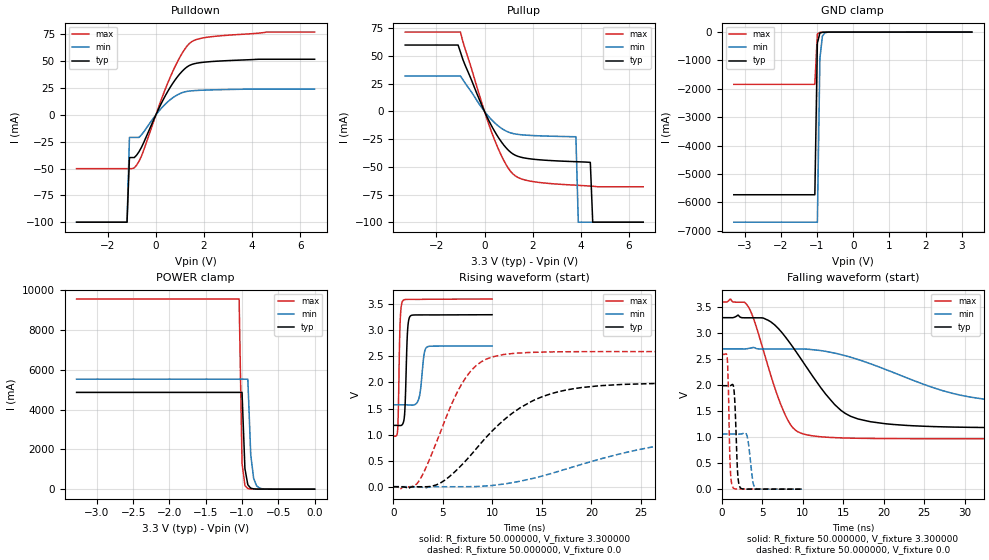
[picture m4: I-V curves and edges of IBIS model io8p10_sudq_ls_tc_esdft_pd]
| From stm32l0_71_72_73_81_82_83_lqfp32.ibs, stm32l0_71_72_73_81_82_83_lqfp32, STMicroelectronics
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|   Model io8p10_sudq_ls_tc_esdft_pd
[Model]  io8p10_sudq_ls_tc_esdft_pd
Model_type I/O
Polarity   Non-Inverting
Enable   Active-Low
Vinl =   0.990000V
Vinh =   2.310000V
Vmeas =  1.650000V
Cref =   50.000000pF
Rref =   100.000000M
Vref =   0.0V
C_comp   2.248300pF   2.207300pF   2.311900pF
[Temperature Range]   25.000000   0.125000k   -40.000000
[Pullup Reference]   3.300000V   2.700000V   3.600000V
[Pulldown Reference]   0.0V   0.0V   0.0V
[POWER Clamp Reference]   3.300000V   2.700000V   3.600000V
[GND Clamp Reference]   0.0V   0.0V   0.0V
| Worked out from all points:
|   slope of the pulldown table from 0 to 0.495 V, typ, clamps not added: 22.6 ohm
|   slope of the pullup table from 0 to 0.495 V, typ, clamps not added: 23.9 ohm
|   GND clamp passes 1 mA (typ) near -0.64 V on its own axis
|   POWER clamp passes 1 mA (typ) near -0.63 V on its own axis
|   rising waveform, R_fixture 50.000000, V_fixture 3.300000: 20-80 % time 208ps typ, 362ps min, 164ps max; typ from 1.18 V to 3.3 V
|   rising waveform, R_fixture 50.000000, V_fixture 0.0: 20-80 % time 6.73ns typ, 13.8ns min, 3.61ns max; typ from 0 V to 1.99 V
|   falling waveform, R_fixture 50.000000, V_fixture 3.300000: 20-80 % time 6.01ns typ, 12.6ns min, 3.29ns max; typ from 3.3 V to 1.18 V
|   falling waveform, R_fixture 50.000000, V_fixture 0.0: 20-80 % time 290ps typ, 459ps min, 228ps max; typ from 1.99 V to 0 V
[Pulldown]
|Voltage   I(typ)   I(min)   I(max)
-3.3V     -100mA     -100mA     -50.11mA
-1.2V     -100mA     -100mA     -50.11mA
-1.1V     -39.8mA    -21mA      -50.11mA
-900mV    -39.8mA    -21mA      -49.43mA
-600mV    -30.26mA   -18.59mA   -38.38mA
500mV     22.11mA    12.28mA    30.06mA
900mV     35.58mA    18.71mA    49.62mA
1.3V      44.74mA    21.88mA    64.23mA
1.7V      48.13mA    22.72mA    70.3mA
2.4V      49.79mA    23.3mA     73.03mA
4.6V      51.8mA     24mA       77.1mA
6.6V      51.8mA     24mA       77.1mA
[Pullup]
|Voltage   I(typ)   I(min)   I(max)
-3.3V     60mA       32mA       71.7mA
-1.1V     60mA       32mA       71.7mA
-1V       53.5mA     32mA       71.7mA
-100mV    4.893mA    2.926mA    6.861mA
400mV     -17.21mA   -9.813mA   -24.69mA
900mV     -32.92mA   -17.72mA   -48.15mA
1.3V      -39.75mA   -20.41mA   -58.47mA
3.8V      -45.36mA   -22.8mA    -66.6mA
3.9V      -45.44mA   -100mA     -66.72mA
4.4V      -46mA      -100mA     -67.4mA
4.5V      -100mA     -100mA     -67.56mA
6.6V      -100mA     -100mA     -68mA
[GND_clamp]
|Voltage   I(typ)   I(min)   I(max)
-3.3V     -5.732A    -6.7A      -1.842A
-1.06V    -5.732A    -6.7A      -1.842A
-990mV    -389.4mA   -6.7A      -68.35mA
-920mV    -32.58mA   -928mA     -10.73mA
-850mV    -6.776mA   -138mA     -6.518mA
-780mV    -3.484mA   -24.13mA   -4.216mA
-570mV    -313uA     -578.6uA   -266.4uA
3.28V     74.9uA     89.13uA    52.44uA
[POWER_clamp]
|Voltage   I(typ)   I(min)   I(max)
-3.28V    4.87A      5.538A     9.569A
-1.04V    4.87A      5.538A     9.569A
-1V       4.87A      5.538A     1.315A
-960mV    1.032A     5.538A     186.5mA
-920mV    222.2mA    5.538A     31.64mA
-880mV    50.73mA    1.734A     9.582mA
-840mV    13.93mA    544.8mA    5.668mA
-800mV    5.556mA    172.7mA    4.276mA
-760mV    3.231mA    55.84mA    3.297mA
-680mV    1.597mA    6.983mA    1.741mA
0V        0A         0A         0A
[Ramp]
| variable   typ   min   max
dV/dt_r  1.19406/6.71991n   0.62628/13.69005n   1.55520/3.60254n
dV/dt_f  1.27332/6.00328n   0.65334/12.50915n   1.57761/3.27787n
R_load = 50.000000
[Rising Waveform]
R_fixture= 50.000000
V_fixture= 3.300000
V_fixture_min= 2.700000
V_fixture_max= 3.600000
|time   V(typ)   V(min)   V(max)
0s        1.176V     1.571V     969.9mV
440.4ps   1.175V     1.571V     1.085V
680.7ps   1.172V     1.571V     3.096V
961ps     1.206V     1.571V     3.567V
1.181ns   1.516V     1.571V     3.59V
1.441ns   2.989V     1.569V     3.593V
1.722ns   3.274V     1.566V     3.593V
2.603ns   3.295V     1.704V     3.593V
3.363ns   3.295V     2.674V     3.595V
9.97ns    3.299V     2.698V     3.599V
[Rising Waveform]
R_fixture= 50.000000
V_fixture= 0.0
V_fixture_min= 0.0
V_fixture_max= 0.0
|time   V(typ)   V(min)   V(max)
0s        8.061uV    -5.324uV   362.7uV
2.503ns   -1.397mV   -3.566mV   85.65mV
4.705ns   66.88mV    -553.3uV   1.021V
6.907ns   416.7mV    -392.7uV   1.97V
8.308ns   714.2mV    2.416mV    2.314V
10.01ns   1.075V     23.02mV    2.491V
14.11ns   1.652V     160.4mV    2.577V
19.02ns   1.902V     429mV      2.591V
31.33ns   1.988V     905.7mV    2.592V
49.85ns   1.99V      1.06V      2.592V
[Falling Waveform]
R_fixture= 50.000000
V_fixture= 3.300000
V_fixture_min= 2.700000
V_fixture_max= 3.600000
|time   V(typ)   V(min)   V(max)
0s        3.299V     2.698V     3.599V
3.303ns   3.296V     2.708V     3.499V
5.706ns   3.25V      2.696V     2.362V
7.508ns   2.994V     2.696V     1.54V
8.609ns   2.767V     2.695V     1.212V
9.81ns    2.496V     2.695V     1.075V
14.71ns   1.515V     2.588V     986.7mV
18.32ns   1.298V     2.414V     975.9mV
30.63ns   1.189V     1.773V     970.2mV
49.85ns   1.176V     1.571V     969.9mV
[Falling Waveform]
R_fixture= 50.000000
V_fixture= 0.0
V_fixture_min= 0.0
V_fixture_max= 0.0
|time   V(typ)   V(min)   V(max)
0s        1.99V      1.06V      2.592V
660.7ps   1.99V      1.06V      2.514V
1.021ns   1.991V     1.06V      450.9mV
1.341ns   2.013V     1.06V      37.89mV
1.582ns   1.722V     1.06V      7.519mV
1.962ns   276.8mV    1.06V      2.37mV
2.262ns   30.57mV    1.06V      2.158mV
3.103ns   696.3uV    1.025V     2.29mV
4.124ns   678.6uV    21.71mV    2.41mV
9.97ns    8.061uV    -5.324uV   362.7uV
